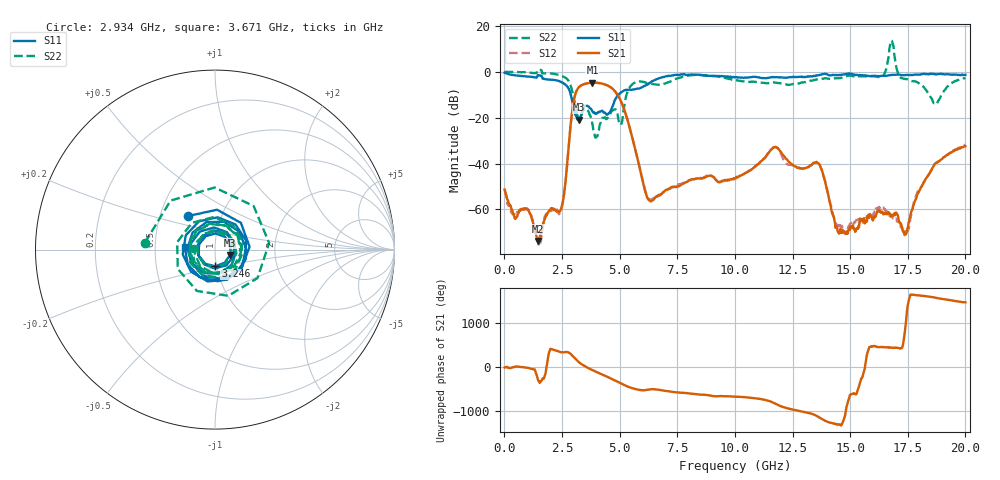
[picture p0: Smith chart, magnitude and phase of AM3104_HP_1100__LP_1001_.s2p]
!Created with skrf (http://scikit-rf.org).
# Hz S RI R 50.0
!freq ReS11 ImS11 ReS21 ImS21 ReS12 ImS12 ReS22 ImS22
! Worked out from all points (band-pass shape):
!   1601 points, 10 MHz to 20 GHz, reference 50 ohm
!   highest |S21| = -4.77 dB at 3.821 GHz (marker M1); lowest = -73.7 dB at 1.447 GHz (marker M2)
!   |S21| within 3 dB of the highest: 3.161 GHz to 4.727 GHz (1.567 GHz wide, 39.7 % of centre)
!   lowest |S11| = -20.9 dB at 3.221 GHz (marker M3), VSWR 1.20, Z = 59.2 - j3.51 ohm
!   |S11| at or under -10 dB: 2.88 GHz to 4.95 GHz (2.07 GHz wide, 52.9 % of centre)
!   |S22| runs from -28.7 to 13.6 dB; largest |S21 - S12| = 0.047
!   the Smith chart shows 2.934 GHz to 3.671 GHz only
!   S11 on the Smith chart (normalised r, x): 2.934 GHz: 0.70, +0.28; 3.246 GHz: 0.99, -0.18; 3.671 GHz: 0.71, +0.02
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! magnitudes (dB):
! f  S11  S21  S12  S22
! 10 MHz  -0.4  -51.3  -51.3  -0.1
! 1.447 GHz  -1.5  -73.7  -73.5  0.8
! 2.471 GHz  -4.5  -59.4  -60.4  -1.8
! 2.934 GHz  -12.4  -17.8  -17.8  -8.1
! 3.221 GHz  -20.9  -6.9  -7.0  -20.3
! 3.246 GHz  -20.7  -6.6  -6.7  -20.3
! 3.346 GHz  -18.6  -5.9  -6.0  -18.8
! 3.671 GHz  -15.5  -4.9  -5.0  -17.9
! 3.821 GHz  -17.3  -4.8  -4.8  -23.0
! 4.945 GHz  -10.1  -10.7  -10.8  -20.8
! 6.169 GHz  -5.8  -54.1  -53.5  -4.9
! 6.682 GHz  -3.0  -53.8  -54.1  -5.7
! 10.01 GHz  -2.5  -46.5  -46.8  -3.7
! 11.73 GHz  -2.4  -32.8  -32.9  -4.7
! 13.34 GHz  -2.1  -40.5  -40.4  -3.9
! 13.73 GHz  -1.3  -41.9  -41.6  -3.3
! 14.55 GHz  -1.4  -69.6  -67.1  -2.8
! 16.38 GHz  -1.8  -61.0  -58.9  -2.2
! 16.68 GHz  -1.6  -61.6  -62.4  7.2
! 17.45 GHz  -1.4  -70.0  -70.4  -3.3
! 18.69 GHz  -1.1  -40.1  -40.2  -13.8
! 20 GHz  -1.3  -32.5  -31.8  -2.8
